| / 7\'7   Xilinx XC18V00 I/O Buffer IBIS File
| \ \   Xilinx Inc.
| / /   2100 Logic Drive
| \_\/.\   San Jose,   CA 95124
[IBIS ver]   2.1
[File name]   xc18v00.ibs
[File Rev]   0.1
[Date]   Nov. 17, 2000
[Source]   Spice netlist
[Notes]   - max/min process data included in this ibis model
   - Created by Joey Jia x4437 on 12/16/1999
|   - Added more package models on 11/17/2000 - SW
[Disclaimer] The data in this model is derived from SPICE simulations
   using modeling information extracted from the target pro-
   cess. While a great deal of care has been take to provide
   information that is accurate, this model is considered
   preliminary as it has not been verified by actual silicon
   measurement. Treat the data in this model as preliminary
   until actual silicon verification is performed.
[Copyright]   Xilinx Inc. All right reserved
|   Component XC18V01_VQ44[VCCIO=2.5]
[Component]   XC18V01_VQ44[VCCIO=2.5]
[Manufacturer]   Xilinx Inc.
[Package]
| variable   typ   min   max
R_pkg   57.000m   54.000m   60.000m
L_pkg   2.260nH   2.100nH   2.430nH
C_pkg   0.275pF   0.260pF   0.290pF
[Pin]  signal_name   model_name   R_pin   L_pin   C_pin
io   iob   IO_00   NA   NA   NA
|   Component XC18V01_VQ44[VCCIO=3.3]
[Component]   XC18V01_VQ44[VCCIO=3.3]
[Manufacturer]   Xilinx Inc.
[Package]
| variable   typ   min   max
R_pkg   57.000m   54.000m   60.000m
L_pkg   2.250nH   2.100nH   2.400nH
C_pkg   0.275pF   0.260pF   0.290pF
[Pin]  signal_name   model_name   R_pin   L_pin   C_pin
io   iob   IO_01   NA   NA   NA
|   Component XC18V01_SO20[VCCIO=2.5]
[Component]   XC18V01_SO20[VCCIO=2.5]
[Manufacturer]   Xilinx Inc.
[Package]
| variable   typ   min   max
R_pkg   54.000m   44.000m   64.000m
L_pkg   2.950nH   2.200nH   3.700nH
C_pkg   0.385pF   0.250pF   0.520pF
[Pin]  signal_name   model_name   R_pin   L_pin   C_pin
io   iob   IO_00   NA   NA   NA
| End [Component] XC18V01_SO20[VCCIO=2.5]
|   Component XC18V01_SO20[VCCIO=3.3]
[Component]   XC18V01_SO20[VCCIO=3.3]
[Manufacturer]   Xilinx Inc.
[Package]
| variable   typ   min   max
R_pkg   54.000m   44.000m   64.000m
L_pkg   2.950nH   2.200nH   3.700nH
C_pkg   0.385pF   0.250pF   0.520pF
[Pin]  signal_name   model_name   R_pin   L_pin   C_pin
io   iob   IO_01   NA   NA   NA
| End [Component] XC18V01_SO20[VCCIO=3.3]
|   Component XC18V01_PC20[VCCIO=2.5]
[Component]   XC18V01_PC20[VCCIO=2.5]
[Manufacturer]   Xilinx Inc.
[Package]
| variable   typ   min   max
R_pkg   53.500m   50.000m   57.000m
L_pkg   3.150nH   2.900nH   3.400nH
C_pkg   0.650pF   0.630pF   0.670pF
[Pin]  signal_name   model_name   R_pin   L_pin   C_pin
io   iob   IO_00   NA   NA   NA
| End [Component] XC18V01_PC20[VCCIO=2.5]
|   Component XC18V01_PC20[VCCIO=3.3]
[Component]   XC18V01_PC20[VCCIO=3.3]
[Manufacturer]   Xilinx Inc.
[Package]
| variable   typ   min   max
R_pkg   53.500m   50.000m   57.000m
L_pkg   3.150nH   2.900nH   3.400nH
C_pkg   0.650pF   0.630pF   0.670pF
[Pin]  signal_name   model_name   R_pin   L_pin   C_pin
io   iob   IO_01   NA   NA   NA
| End [Component] XC18V01_PC20[VCCIO=3.3]
|   Component XC18V256_VQ44[VCCIO=2.5]
[Component]   XC18V256_VQ44[VCCIO=2.5]
[Manufacturer]   Xilinx Inc.
[Package]
| variable   typ   min   max
R_pkg   57.000m   54.000m   60.000m
L_pkg   2.260nH   2.100nH   2.430nH
C_pkg   0.275pF   0.260pF   0.290pF
[Pin]  signal_name   model_name   R_pin   L_pin   C_pin
io   iob   IO_00   NA   NA   NA
| End [Component] XC18V256_VQ44[VCCIO=2.5]
|   Component XC18V256_VQ44[VCCIO=3.3]
[Component]   XC18V256_VQ44[VCCIO=3.3]
[Manufacturer]   Xilinx Inc.
[Package]
| variable   typ   min   max
R_pkg   57.000m   54.000m   60.000m
L_pkg   2.260nH   2.100nH   2.430nH
C_pkg   0.275pF   0.260pF   0.290pF
[Pin]  signal_name   model_name   R_pin   L_pin   C_pin
io   iob   IO_01   NA   NA   NA
| End [Component] XC18V256_VQ44[VCCIO=3.3]
|   Component XC18V256_SO20[VCCIO=2.5]
[Component]   XC18V256_SO20[VCCIO=2.5]
[Manufacturer]   Xilinx Inc.
[Package]
| variable   typ   min   max
R_pkg   54.000m   44.000m   64.000m
L_pkg   2.950nH   2.200nH   3.700nH
C_pkg   0.385pF   0.250pF   0.520pF
[Pin]  signal_name   model_name   R_pin   L_pin   C_pin
io   iob   IO_00   NA   NA   NA
| End [Component] XC18V256_SO20[VCCIO=2.5]
|   Component XC18V256_SO20[VCCIO=3.3]
[Component]   XC18V256_SO20[VCCIO=3.3]
[Manufacturer]   Xilinx Inc.
[Package]
| variable   typ   min   max
R_pkg   54.000m   44.000m   64.000m
L_pkg   2.950nH   2.200nH   3.700nH
C_pkg   0.385pF   0.250pF   0.520pF
[Pin]  signal_name   model_name   R_pin   L_pin   C_pin
io   iob   IO_01   NA   NA   NA
| End [Component] XC18V256_SO20[VCCIO=3.3]
|   Component XC18V256_PC20[VCCIO=2.5]
[Component]   XC18V256_PC20[VCCIO=2.5]
[Manufacturer]   Xilinx Inc.
[Package]
| variable   typ   min   max
R_pkg   53.500m   50.000m   57.000m
L_pkg   3.150nH   2.900nH   3.400nH
C_pkg   0.650pF   0.630pF   0.670pF
[Pin]  signal_name   model_name   R_pin   L_pin   C_pin
io   iob   IO_00   NA   NA   NA
| End [Component] XC18V256_PC20[VCCIO=2.5]
|   Component XC18V256_PC20[VCCIO=3.3]
[Component]   XC18V256_PC20[VCCIO=3.3]
[Manufacturer]   Xilinx Inc.
[Package]
| variable   typ   min   max
R_pkg   53.500m   50.000m   57.000m
L_pkg   3.150nH   2.900nH   3.400nH
C_pkg   0.650pF   0.630pF   0.670pF
[Pin]  signal_name   model_name   R_pin   L_pin   C_pin
io   iob   IO_01   NA   NA   NA
| End [Component] XC18V256_PC20[VCCIO=3.3]
|   Component XC18V512_VQ44[VCCIO=2.5]
[Component]   XC18V512_VQ44[VCCIO=2.5]
[Manufacturer]   Xilinx Inc.
[Package]
| variable   typ   min   max
R_pkg   57.000m   54.000m   60.000m
L_pkg   2.260nH   2.100nH   2.430nH
C_pkg   0.275pF   0.260pF   0.290pF
[Pin]  signal_name   model_name   R_pin   L_pin   C_pin
io   iob   IO_00   NA   NA   NA
| End [Component] XC18V512_VQ44[VCCIO=2.5]
|   Component XC18V512_VQ44[VCCIO=3.3]
[Component]   XC18V512_VQ44[VCCIO=3.3]
[Manufacturer]   Xilinx Inc.
[Package]
| variable   typ   min   max
R_pkg   57.000m   54.000m   60.000m
L_pkg   2.260nH   2.100nH   2.430nH
C_pkg   0.275pF   0.260pF   0.290pF
[Pin]  signal_name   model_name   R_pin   L_pin   C_pin
io   iob   IO_01   NA   NA   NA
| End [Component] XC18V512_VQ44[VCCIO=3.3]
|   Component XC18V512_SO20[VCCIO=2.5]
[Component]   XC18V512_SO20[VCCIO=2.5]
[Manufacturer]   Xilinx Inc.
[Package]
| variable   typ   min   max
R_pkg   54.000m   44.000m   64.000m
L_pkg   2.950nH   2.200nH   3.700nH
C_pkg   0.385pF   0.250pF   0.520pF
[Pin]  signal_name   model_name   R_pin   L_pin   C_pin
io   iob   IO_00   NA   NA   NA
| End [Component] XC18V512_SO20[VCCIO=2.5]
|   Component XC18V512_SO20[VCCIO=3.3]
[Component]   XC18V512_SO20[VCCIO=3.3]
[Manufacturer]   Xilinx Inc.
[Package]
| variable   typ   min   max
R_pkg   54.000m   44.000m   64.000m
L_pkg   2.950nH   2.200nH   3.700nH
C_pkg   0.385pF   0.250pF   0.520pF
[Pin]  signal_name   model_name   R_pin   L_pin   C_pin
io   iob   IO_01   NA   NA   NA
| End [Component] XC18V512_SO20[VCCIO=3.3]
|   Component XC18V512_PC20[VCCIO=2.5]
[Component]   XC18V512_PC20[VCCIO=2.5]
[Manufacturer]   Xilinx Inc.
[Package]
| variable   typ   min   max
R_pkg   53.500m   50.000m   57.000m
L_pkg   3.150nH   2.900nH   3.400nH
C_pkg   0.650pF   0.630pF   0.670pF
[Pin]  signal_name   model_name   R_pin   L_pin   C_pin
io   iob   IO_00   NA   NA   NA
| End [Component] XC18V512_PC20[VCCIO=2.5]
|   Component XC18V512_PC20[VCCIO=3.3]
[Component]   XC18V512_PC20[VCCIO=3.3]
[Manufacturer]   Xilinx Inc.
[Package]
| variable   typ   min   max
R_pkg   53.500m   50.000m   57.000m
L_pkg   3.150nH   2.900nH   3.400nH
C_pkg   0.650pF   0.630pF   0.670pF
[Pin]  signal_name   model_name   R_pin   L_pin   C_pin
io   iob   IO_01   NA   NA   NA
| End [Component] XC18V512_PC20[VCCIO=3.3]
|   Component XC18V02_VQ44[VCCIO=2.5]
[Component]   XC18V02_VQ44[VCCIO=2.5]
[Manufacturer]   Xilinx Inc.
[Package]
| variable   typ   min   max
R_pkg   48.500m   46.000m   51.000m
L_pkg   1.900nH   1.800nH   2.000nH
C_pkg   0.235pF   0.220pF   0.250pF
[Pin]  signal_name   model_name   R_pin   L_pin   C_pin
io   iob   IO_00   NA   NA   NA
| End [Component] XC18V02_VQ44[VCCIO=2.5]
|   Component XC18V02_VQ44[VCCIO=3.3]
[Component]   XC18V02_VQ44[VCCIO=3.3]
[Manufacturer]   Xilinx Inc.
[Package]
| variable   typ   min   max
R_pkg   48.500m   46.000m   51.000m
L_pkg   1.900nH   1.800nH   2.000nH
C_pkg   0.235pF   0.220pF   0.250pF
[Pin]  signal_name   model_name   R_pin   L_pin   C_pin
io   iob   IO_01   NA   NA   NA
| End [Component] XC18V02_VQ44[VCCIO=3.3]
|   Component XC18V02_PC44[VCCIO=2.5]
[Component]   XC18V02_PC44[VCCIO=2.5]
[Manufacturer]   Xilinx Inc.
[Package]
| variable   typ   min   max
R_pkg   67.500m   66.000m   69.000m
L_pkg   3.910nH   3.550nH   4.260nH
C_pkg   0.890pF   0.790pF   1.000pF
[Pin]  signal_name   model_name   R_pin   L_pin   C_pin
io   iob   IO_00   NA   NA   NA
| End [Component] XC18V02_PC44[VCCIO=2.5]
|   Component XC18V02_PC44[VCCIO=3.3]
[Component]   XC18V02_PC44[VCCIO=3.3]
[Manufacturer]   Xilinx Inc.
[Package]
| variable   typ   min   max
R_pkg   67.500m   66.000m   69.000m
L_pkg   3.910nH   3.550nH   4.260nH
C_pkg   0.890pF   0.790pF   1.000pF
[Pin]  signal_name   model_name   R_pin   L_pin   C_pin
io   iob   IO_01   NA   NA   NA
| End [Component] XC18V02_PC44[VCCIO=3.3]
|   Component XC18V04_VQ44[VCCIO=2.5]
[Component]   XC18V04_VQ44[VCCIO=2.5]
[Manufacturer]   Xilinx Inc.
[Package]
| variable   typ   min   max
R_pkg   48.500m   46.000m   51.000m
L_pkg   1.900nH   1.800nH   2.000nH
C_pkg   0.235pF   0.220pF   0.250pF
[Pin]  signal_name   model_name   R_pin   L_pin   C_pin
io   iob   IO_00   NA   NA   NA
| End [Component] XC18V04_VQ44[VCCIO=2.5]
|   Component XC18V04_VQ44[VCCIO=3.3]
[Component]   XC18V04_VQ44[VCCIO=3.3]
[Manufacturer]   Xilinx Inc.
[Package]
| variable   typ   min   max
R_pkg   48.500m   46.000m   51.000m
L_pkg   1.900nH   1.800nH   2.000nH
C_pkg   0.235pF   0.220pF   0.250pF
[Pin]  signal_name   model_name   R_pin   L_pin   C_pin
io   iob   IO_01   NA   NA   NA
| End [Component] XC18V04_VQ44[VCCIO=3.3]
|   Component XC18V04_PC44[VCCIO=2.5]
[Component]   XC18V04_PC44[VCCIO=2.5]
[Manufacturer]   Xilinx Inc.
[Package]
| variable   typ   min   max
R_pkg   67.500m   66.000m   69.000m
L_pkg   3.910nH   3.550nH   4.260nH
C_pkg   0.890pF   0.790pF   1.000pF
[Pin]  signal_name   model_name   R_pin   L_pin   C_pin
io   iob   IO_00   NA   NA   NA
| End [Component] XC18V04_PC44[VCCIO=2.5]
|   Component XC18V04_PC44[VCCIO=3.3]
[Component]   XC18V04_PC44[VCCIO=3.3]
[Manufacturer]   Xilinx Inc.
[Package]
| variable   typ   min   max
R_pkg   67.500m   66.000m   69.000m
L_pkg   3.910nH   3.550nH   4.260nH
C_pkg   0.890pF   0.790pF   1.000pF
[Pin]  signal_name   model_name   R_pin   L_pin   C_pin
io   iob   IO_01   NA   NA   NA
| End [Component] XC18V04_PC44[VCCIO=3.3]
|   Component XC18V04_PQ44[VCCIO=2.5]
[Component]   XC18V04_PQ44[VCCIO=2.5]
[Manufacturer]   Xilinx Inc.
[Package]
| variable   typ   min   max
R_pkg   53.500m   51.000m   56.000m
L_pkg   2.100nH   2.000nH   2.200nH
C_pkg   0.260pF   0.240pF   0.280pF
[Pin]  signal_name   model_name   R_pin   L_pin   C_pin
io   iob   IO_00   NA   NA   NA
| End [Component] XC18V04_PQ44[VCCIO=2.5]
|   Component XC18V04_PQ44[VCCIO=3.3]
[Component]   XC18V04_PQ44[VCCIO=3.3]
[Manufacturer]   Xilinx Inc.
[Package]
| variable   typ   min   max
R_pkg   53.500m   51.000m   56.000m
L_pkg   2.100nH   2.000nH   2.200nH
C_pkg   0.260pF   0.240pF   0.280pF
[Pin]  signal_name   model_name   R_pin   L_pin   C_pin
io   iob   IO_01   NA   NA   NA
| End [Component] XC18V04_PQ44[VCCIO=3.3]
| Models and submodels in the file (2): IO_00 (I/O), IO_01 (I/O)
